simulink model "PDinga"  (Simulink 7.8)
settings: Solver=ode3  StartTime=0.0  StopTime=100  FixedStep=0.1  RelTol=1e-3
undefined symbols (not defined in the file or in its folder): deg, kg, m, N, s
libraries: mblibv1 x8, simulink x3

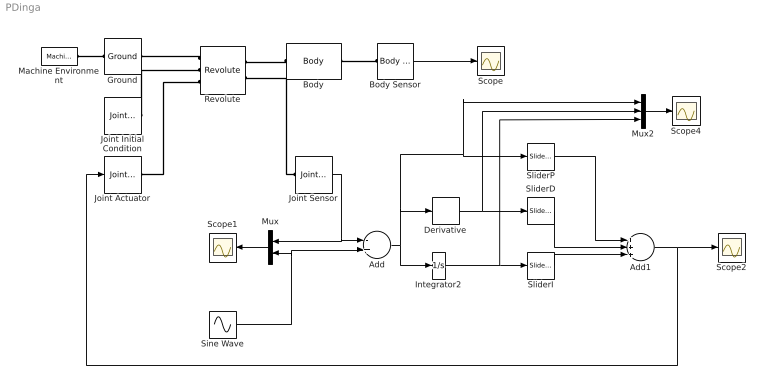
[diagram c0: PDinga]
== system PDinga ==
  Add : Sum  Inputs=-+
  Add1 : Sum  Inputs=+++
  Body : mblibv1/Bodies/Body  LConnTagsString=CS1  RConnTagsString=CS2  UpdateFromCAD=off  DialogClass=MechanicalBodyBlock  Mass=1  MassUnits=kg  InertiaUnits=kg*m^2  Inertia=eye(3)  Shape=Cylinder  ShapeDims=[1 1]  ShapeUnits=m  ShapeUse=false  Density=1  DensityUnits=kg/m^3  DensityUse=false  GraphicsMode=MACHINE_DEFAULT  BodyColorSelMode=MACHINE_DEFAULT  BodyColor=[1 0 0]  AttachedToCS=CG  CG=Left$CG$[0 -0.5 0]$WORLD$WORLD$m$[0 0 0]$Euler X-Y-Z$deg$WORLD$false$none  WorkingFrames=Left$CS1$[0 0.5 0]$CG$CG$m$[0 0 0]$Euler X-Y-Z$deg$WORLD$true$none#Right$CS2$[0 -0.5 0]$CG$CG$m$[0 0 0]$Euler X-Y-Z$deg$WORLD$true$none  CGPos=[0 -0.5 0]  CGRot=[0 0 0]  CS0Pos=[]  CS0Rot=[]  CS1Pos=[0 0.5 0]  CS1Rot=[0 0 0]  CS2Pos=[0 -0.5 0]  CS2Rot=[0 0 0]  CS3Pos=[]  CS3Rot=[]  CS4Pos=[]  CS4Rot=[]  CS5Pos=[]  CS5Rot=[]  CS6Pos=[]  CS6Rot=[]  CS7Pos=[]  CS7Rot=[]  CS8Pos=[]  CS8Rot=[]  CS9Pos=[]  CS9Rot=[]  CS10Pos=[]  CS10Rot=[]  CS11Pos=[]  CS11Rot=[]  CS12Pos=[]  CS12Rot=[]  CS13Pos=[]  CS13Rot=[]  CS14Pos=[]  CS14Rot=[]  CS15Pos=[]  CS15Rot=[]  CS16Pos=[]  CS16Rot=[]  CS17Pos=[]  CS17Rot=[]  CS18Pos=[]  CS18Rot=[]  CS19Pos=[]  CS19Rot=[]  CS20Pos=[]  CS20Rot=[]
  Body Sensor : mblibv1/Sensors &  Actuators/Body Sensor  UpdateFromCAD=off  PhysicalDomain=Mechanical  PortType=blob  Muxed=on  Pose=off  Angle=on  AngleUnits=deg  ArcVelocity=off  ArcVelocityUnits=deg/s  ArcAcceleration=off  ArcAccelerationUnits=deg/s^2  CoordPosition=on  CoordPositionUnits=m  Velocity=off  VelocityUnits=m/s  Acceleration=off  AccelerationUnits=m/s^2  Quaternion=on  QuaternionDT=off  QuaternionDDT=off  QuaternionUnits=off  OutputVector=[1]  ActiveIO=on  Width=3  DialogClass=MechanicalSensorBlock  ReferenceFrame=Absolute (World)
  Derivative : Derivative
  Ground : mblibv1/Bodies/Ground  UpdateFromCAD=off  LeftPortType=env  RightPortType=workingframe  PhysicalDomain=Mechanical  DialogClass=GroundBlock  CoordPosition=[0 0 0]  CoordPositionUnits=m  StateVectorMgrId=0  MachineId=[1 0]  ShowEnvPort=on
  Integrator2 : Integrator
  Joint Actuator : mblibv1/Sensors &  Actuators/Joint Actuator  UpdateFromCAD=off  PhysicalDomain=Mechanical  PortType=blob  ActuationStyle=Force  AngleUnits=deg  ArcVelocityUnits=deg/s  ArcAccelerationUnits=deg/s^2  CoordPositionUnits=m  VelocityUnits=m/s  AccelerationUnits=m/s^2  ForceUnits=N  TorqueUnits=N*m  ActiveIO=on  Width=1  DialogClass=MechanicalActuatorBlock  Primitive=R1  ReferenceFrame=Absolute (World)
  Joint Initial Condition : mblibv1/Sensors &  Actuators/Joint Initial Condition  UpdateFromCAD=off  LeftPortType=blob  RightPortType=blob  PhysicalDomain=mechanical  DialogClass=InitialConditionBlock  InitialConditions=P1$false$0$m$deg$0$m/s$deg/s#P2$false$0$m$deg$0$m/s$deg/s#P3$false$0$m$deg$0$m/s$deg/s#R1$true$0$m$rad$0$m/s$rad/s#R2$false$0$m$deg$0$m/s$deg/s#R3$false$0$m$deg$0$m/s$deg/s#S$false$0$m$deg$0$m/s$deg/s  P1PIC=0  P1VIC=0  P2PIC=0  P2VIC=0  P3PIC=0  P3VIC=0  R1PIC=0  R1VIC=0  R2PIC=0  R2VIC=0  R3PIC=0  R3VIC=0  SPIC=0  SVIC=0
  Joint Sensor : mblibv1/Sensors &  Actuators/Joint Sensor  UpdateFromCAD=off  PhysicalDomain=Mechanical  PortType=blob  Muxed=on  Pose=off  Angle=on  AngleUnits=deg  ArcVelocity=off  ArcVelocityUnits=deg/s  ArcAcceleration=off  ArcAccelerationUnits=deg/s^2  CoordPosition=on  CoordPositionUnits=m  Velocity=off  VelocityUnits=m/s  Acceleration=off  AccelerationUnits=m/s^2  Quaternion=on  QuaternionDT=off  QuaternionDDT=off  QuaternionUnits=off  OutputVector=[1]  ActiveIO=on  Width=1  DialogClass=MechanicalSensorBlock  Primitive=R1  Force=off  ForceUnits=N  Torque=off  TorqueUnits=N*m  ReferenceFrame=Absolute (World)  ReactionSensedSide=Base  ReactionReferenceFrame=Absolute (World)  ReactionForce=off  ReactionForceUnits=N  ReactionMoment=off  ReactionMomentUnits=N*m
  Machine Environment : mblibv1/Bodies/Machine Environment  Tag=Factory ground  PortType=env  PhysicalDomain=Mechanical  DialogTemplateClass=MECH.MachineEnvironment  SyncWhenCopied=off  Gravity=[0 -9.81 0]  GravityUnits=m/s^2  GravityAsSignal=off  Dimensionality=Auto-detect  AnalysisType=Forward dynamics  LinearAssemblyTolerance=1e-3  LinearAssemblyToleranceUnits=m  AngularAssemblyTolerance=1e-3  AngularAssemblyToleranceUnits=rad  ConstraintSolverType=Stabilizing  ConstraintRelTolerance=1e-4  ConstraintAbsTolerance=1e-4  UseRobustSingularityHandling=off  RedundancyAnalysisToleranceType=Automatically select tolerance  RedundancyAnalysisTolerance=1e-14  StatePerturbationType=Fixed  PerturbationSize=1e-5  VisualizeMachine=on  BodyVisualizationType=Use model default body geometries  BodyColorSelMode=Use model default  DefaultBodyColor=[1 0 0]
  Mux : Mux  Inputs=2
  Mux2 : Mux  Inputs=3
  Revolute : mblibv1/Joints/Revolute  LConnTagsString=__newl0|SA1|SA2  RConnTagsString=__newr0|SA1  UpdateFromCAD=off  NumSAPorts=3  CutJoint=off  MarkAsCut=off  Primitives=prismatic  PrimitiveProps=R1$World$[0 0 1]$revolute  DialogClass=JointBlock  R1Axis=[0 0 1]
  Scope{,1..2,4} (4 alike) : Scope
  Sine Wave : Sin  Amplitude=15  Frequency=0.1  SampleTime=0
  SliderD : simulink/Math Operations/Slider Gain  low=0  gain=0.1  high=10
  SliderI : simulink/Math Operations/Slider Gain  low=0  gain=0.1  high=10
  SliderP : simulink/Math Operations/Slider Gain  low=0  gain=4  high=20
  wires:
  Body Sensor/1 -> Scope/1
  Joint Sensor/1 -> Add/1, Mux/1
  SliderP/1 -> Add1/1
  SliderD/1 -> Add1/2
  Add1/1 -> Scope2/1, Joint Actuator/1
  Mux/1 -> Scope1/1
  Integrator2/1 -> SliderI/1, Mux2/3
  SliderI/1 -> Add1/3
  Add/1 -> Derivative/1, SliderP/1, Mux2/1, Integrator2/1
  Derivative/1 -> SliderD/1, Mux2/2
  Sine Wave/1 -> Add/2, Mux/2
  Mux2/1 -> Scope4/1
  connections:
  Machine Environment/RConn1 -- Ground/LConn1
  Revolute/LConn1 -- Ground/RConn1
  Body/LConn1 -- Revolute/RConn1
  Body Sensor/LConn1 -- Body/RConn1
  Joint Initial Condition/RConn1 -- Revolute/LConn2
  Joint Actuator/RConn1 -- Revolute/LConn3
  Joint Sensor/LConn1 -- Revolute/RConn2
